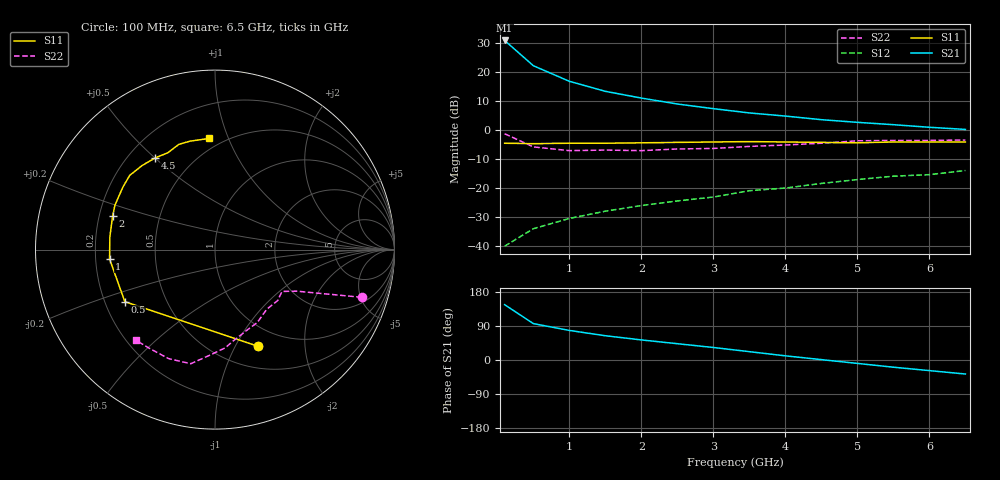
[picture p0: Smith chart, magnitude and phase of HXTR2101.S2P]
! HXTR-2101  (2N6679) Common Emitter
! Vce=15V  Ic=25mA
# ghz s ma r 50
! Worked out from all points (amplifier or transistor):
!   14 points, 100 MHz to 6.5 GHz, reference 50 ohm
!   highest |S21| = 30.8 dB at 100 MHz (marker M1)
!   |S21| within 3 dB of that: start of sweep to 237.8 MHz
!   unconditionally stable (mu >= 1): 736.7 MHz to 3.929 GHz
!   at 1 GHz: K = 1.14, MAG = 21.3 dB, |S12| = -30.5 dB
!   at 3.5 GHz: K = 1.02, MAG = 12.5 dB, |S12| = -20.9 dB
!   at 6.5 GHz: K = 0.57, MSG = 7.1 dB, |S12| = -14.0 dB
!   S11 on the Smith chart (normalised r, x): 100 MHz: 0.75, -1.24; 500 MHz: 0.28, -0.25; 1 GHz: 0.26, -0.04; 2 GHz: 0.26, +0.15; 4.5 GHz: 0.31, +0.50; 6.5 GHz: 0.42, +0.85
0.1  0.59 -66.0  34.6 146.0  0.01 69.0  0.86 -18.0
0.5  0.58 -150.0  12.7 96.0  0.02 44.0  0.51 -27.0
1  0.59 -175.0  6.86 78.0  0.03 51.0  0.44 -32.0
1.5  0.59 173.0  4.61 64.0  0.04 55.0  0.45 -39.0
2  0.6 162.0  3.53 53.0  0.05 55.0  0.44 -49.0
2.5  0.61 156.0  2.79 43.0  0.06 55.0  0.47 -60.0
3  0.62 146.0  2.32 33.0  0.07 56.0  0.48 -67.0
3.5  0.63 139.0  1.96 22.0  0.09 53.0  0.52 -79.0
4  0.62 131.0  1.73 11.0  0.1 50.0  0.55 -84.0
4.5  0.61 123.0  1.5 1.0  0.12 48.0  0.59 -93.0
5  0.6 116.0  1.35 -9.0  0.14 44.0  0.65 -102.0
5.5  0.62 109.0  1.23 -19.0  0.16 36.0  0.66 -113.0
6  0.62 103.0  1.11 -28.0  0.17 32.0  0.66 -123.0
6.5  0.62 93.0  1.02 -37.0  0.2 28.0  0.67 -131.0
